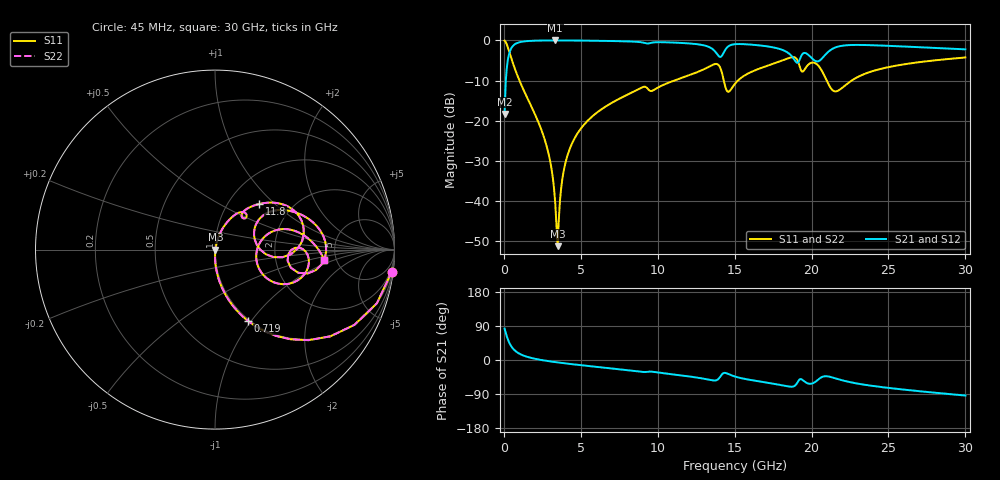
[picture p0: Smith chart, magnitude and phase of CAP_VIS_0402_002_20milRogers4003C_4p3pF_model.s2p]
! S-parameter model data by Modelithics Inc.  support@modelithics.com  813-866-6335  Tampa FL USA
! S-Parameter data specifications:
! Substrate: 20-mil Rogers 4003C, substrate thickness, H=0.508mm, Dielectric constant, Er=3.75
! PCB Mounting Pad Footprint: Pad width, PadW=0.50mm , Pad length, PadL=0.50mm , Pad gap, PadG (edge-to-edge)=0.40mm , Reference planes=1.4mm apart
! Created Wed Nov 18 12:47:37 2015
# hz S ma R 50
! 2 Port Network Data from SP1.SP block
! freq  magS11  angS11  magS21  angS21  magS12  angS12  magS22  angS22
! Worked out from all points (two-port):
!   401 points, 45 MHz to 30 GHz, reference 50 ohm
!   highest |S21| = -0.02 dB at 3.34 GHz (marker M1); lowest = -18.3 dB at 45 MHz (marker M2)
!   |S21| within 3 dB of the highest: 365.3 MHz to 13.78 GHz (13.42 GHz wide, 190 % of centre); 21.04 GHz to end of sweep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
!   lowest |S11| = -51.2 dB at 3.49 GHz (marker M3), VSWR 1.01, Z = 50.3 + j0.0196 ohm
!   |S11| at or under -10 dB: 1.009 GHz to 11.08 GHz (10.07 GHz wide, 167 % of centre); 14.29 GHz to 15.21 GHz (919 MHz wide, 6.23 % of centre); 20.98 GHz to 22.61 GHz (1.627 GHz wide, 7.46 % of centre)
!   |S22| runs from -51.2 to -0.1 dB; largest |S21 - S12| = 0
!   S11 on the Smith chart (normalised r, x): 45 MHz: 1, -16; 719 MHz: 0.98, -0.97; 11.8 GHz: 1.38, +0.80; 30 GHz: 4.02, -0.73
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4.5e7  0.9926 -7.1  0.1216 82.9  0.1216 82.9  0.9926 -7.1
3.4455e8  0.7256 -44.1  0.6874 45.9  0.6874 45.9  0.7256 -44.1
7.189875e8  0.439 -65.1  0.8973 24.7  0.8973 24.7  0.439 -65.1
2.74095e9  0.0512 -89.4  0.9962 -2.0  0.9962 -2.0  0.0512 -89.4
3.115388e9  0.0238 -88.2  0.9971 -4.3  0.9971 -4.3  0.0238 -88.2
3.34005e9  0.009226 -78.9  0.9972 -5.6  0.9972 -5.6  0.009226 -78.9
3.489825e9  0.002746 4.1  0.9972 -6.4  0.9972 -6.4  0.002746 4.1
4.088925e9  0.03466 75.7  0.9963 -9.4  0.9963 -9.4  0.03466 75.7
5.062462e9  0.08258 73.8  0.9931 -13.9  0.9931 -13.9  0.08258 73.8
1.007992e10  0.263 53.3  0.9497 -33.5  0.9497 -33.5  0.263 53.3
1.180234e10  0.3542 45.9  0.9225 -42.1  0.9225 -42.1  0.3542 45.9
1.38243e10  0.509 14.6  0.6893 -53.2  0.6893 -53.2  0.509 14.6
1.449829e10  0.2343 6.7  0.813 -35.3  0.813 -35.3  0.2343 6.7
1.50225e10  0.2886 33.8  0.8963 -43.6  0.8963 -43.6  0.2886 33.8
1.726912e10  0.4938 24.8  0.8332 -60.9  0.8332 -60.9  0.4938 24.8
1.869199e10  0.6156 4.3  0.6421 -70.5  0.6421 -70.5  0.6156 4.3
1.936598e10  0.4092 -8.7  0.6594 -51.4  0.6594 -51.4  0.4092 -8.7
2.003996e10  0.5281 -7.7  0.5946 -62.0  0.5946 -62.0  0.5281 -7.7
2.063906e10  0.4279 -26.8  0.5848 -45.6  0.5848 -45.6  0.4279 -26.8
2.153771e10  0.2316 -6.5  0.8146 -48.3  0.8146 -48.3  0.2316 -6.5
2.505742e10  0.4669 12.4  0.8538 -73.9  0.8538 -73.9  0.4669 12.4
3e10  0.6124 -5.3  0.7727 -93.8  0.7727 -93.8  0.6124 -5.3
